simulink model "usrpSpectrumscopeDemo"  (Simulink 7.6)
settings: Solver=FixedStepDiscrete  StartTime=0.0  StopTime=inf  RelTol=1e-3
PostLoadFcn:
  | set_param([gcs,'/usrp_helper'],'firmware','');
  | set_param([gcs,'/usrp_helper'],'bitstream','')
undefined symbols (not defined in the file or in its folder): Bit, Channels, Complex, dBW, Fs, get, Hertz, INT16, kB, kSps, Mbit, N, S, s
libraries: simulink x2, usrp_GPP x2, dspsnks4 x1

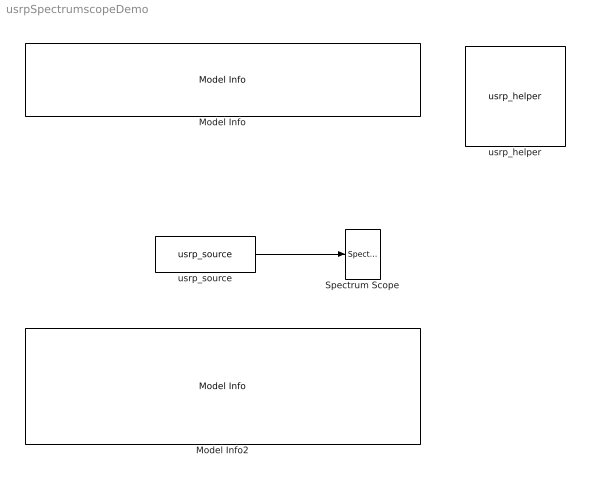
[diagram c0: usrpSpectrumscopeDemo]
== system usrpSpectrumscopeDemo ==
  Model Info : simulink/Model-Wide Utilities/Model Info  SystemSampleTime=-1  InitialBlockCM=None  BlockCM=None  Frame=on  DisplayStringWithTags=USRP Spectrum Scope Demo  HorizontalTextAlignment=Center  LeftAlignmentValue=0.5  SourceBlockDiagram=usrpSpectrumscopeDemo  TagMaxNumber=20
  Model Info2 : simulink/Model-Wide Utilities/Model Info  SystemSampleTime=-1  InitialBlockCM=None  BlockCM=None  Frame=on  DisplayStringWithTags=|  HorizontalTextAlignment=Center  LeftAlignmentValue=0.5  SourceBlockDiagram=usrpSpectrumscopeDemo  TagMaxNumber=20
      | This model samples a signal at 27 MHz and
      | displays it FFT in a Spectrum Scope.
      | 
      | Change the frequency in the usrp_source
      | block to match one supported by your
      | installed daugtherboards.
  Spectrum Scope : dspsnks4/Spectrum Scope  DialogController=dspdialog.SpectrumScope  DialogControllerArgs=DataTag0  SystemSampleTime=-1  ScopeProperties=on  Domain=Frequency  HorizSpan=1  UseBuffer=off  BufferSize=128  Overlap=64  inpFftLenInherit=off  FFTlength=128  numAvg=2  DisplayProperties=off  AxisGrid=on  Memory=off  FrameNumber=on  AxisLegend=off  AxisZoom=off  OpenScopeAtSimStart=on  OpenScopeImmediately=off  FigPos=get(0,'defaultfigureposition')  AxisProperties=off  XUnits=Hertz  XRange=[-Fs/2...Fs/2]  XDisplay=0  InheritXIncr=on  XIncr=1.0  XLabel=Samples  XLimit=Auto  YUnits=dBW/Hertz  XMax=1  XMin=0  YLabel=Magnitude-squared, dB  LineProperties=off  wintypeSpecScope=Hann  RsSpecScope=50  betaSpecScope=5  winsampSpecScope=Periodic  XAxisParamsVer=6.8
  usrp_helper : usrp_GPP/usrp_helper  usrp_number=0  serial_number=S/N: 4556d9c1.  daughterboards_rx=RX A: Flex 2400 Rx, RX B: WBX NG RX,  daughterboards_tx=TX A: Flex 2400 Tx, TX B: WBX NG TX.  usb_block_size=0  usb_nblocks=0  firmware=C:\Users\nagel\Documents\sff_sdr\Simulink-USRP\simulink-usrp_2.1.0\firmware\rev4\std.ihx  bitstream=C:\Users\nagel\Documents\sff_sdr\Simulink-USRP\simulink-usrp_2.1.0\firmware\rev4\std_2rxhb_2tx.rbf  sample_time_factor=1
  usrp_source : usrp_GPP/usrp_source  usrp_number=0  serial_number=S/N: 4556d9c1.  decimation=256  sample_width=16 Bit  sampling_rate_and_bandwidth=1 Channels: 250 kSps, 976.563 kB/s, 7.62939 Mbit/s.  vector_length=128  sideA_subdev1_tab_=0  sideA_subdev1_subdevice=Flex 2400 Rx  sideA_subdev1_datatype=INT16 Complex  sideA_subdev1_frequency_range=Min: 2.3 GHz, Max: 2.9 GHz.  sideA_subdev1_frequency_port=off  sideA_subdev1_frequency=2.4e9  sideA_subdev1_gain_range=Min: 0 dB, Max: 90 dB, Step Size: 0.05 dB.  sideA_subdev1_gain=0  sideA_subdev1_antenna=Not applicable  sideA_subdev2_tab_=0  sideA_subdev2_subdevice=Not available.  sideA_subdev2_datatype=Disabled  sideA_subdev2_frequency_range=Unknown.  sideA_subdev2_frequency_port=off  sideA_subdev2_frequency=0  sideA_subdev2_gain_range=Unknown.  sideA_subdev2_gain=0  sideB_subdev1_tab_=0  sideB_subdev1_subdevice=WBX NG RX  sideB_subdev1_datatype=Disabled  sideB_subdev1_frequency_range=Min: 68.75 MHz, Max: 2.2 GHz.  sideB_subdev1_frequency_port=off  sideB_subdev1_frequency=0  sideB_subdev1_gain_range=Min: 0 dB, Max: 50.5 dB, Step Size: 0.05 dB.  sideB_subdev1_gain=0  sideB_subdev1_antenna=Not applicable  sideB_subdev2_subdevice=Not available.  sideB_subdev2_datatype=Disabled  sideB_subdev2_frequency_range=Unknown.  sideB_subdev2_frequency_port=off  sideB_subdev2_frequency=0  sideB_subdev2_gain_range=Unknown.  sideB_subdev2_gain=0
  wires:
  usrp_source/1 -> Spectrum Scope/1
